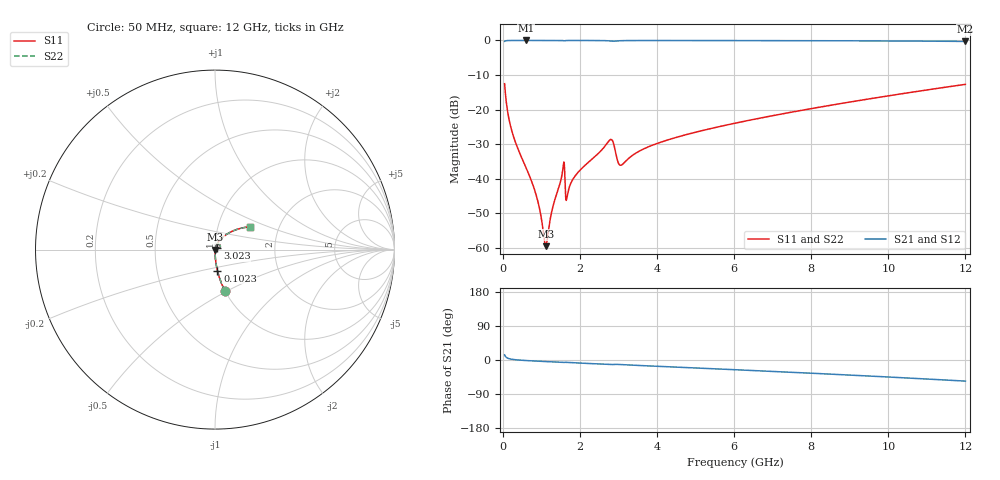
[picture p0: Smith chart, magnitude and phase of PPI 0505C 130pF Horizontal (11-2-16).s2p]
# MHz S MA R 50
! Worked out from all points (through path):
!   1601 points, 50 MHz to 12 GHz, reference 50 ohm
!   highest |S21| = -0.01 dB at 602.7 MHz (marker M1); lowest = -0.3 dB at 12 GHz (marker M2)
!   group delay of S21, straight-line fit = 13 ps
!   lowest |S11| = -59.5 dB at 1.118 GHz (marker M3), VSWR 1.00, Z = 50.1 - j0.00725 ohm
!   |S11| at or under -10 dB: start of sweep to end of sweep
!   |S22| runs from -59.5 to -12.5 dB; largest |S21 - S12| = 0
!   S11 on the Smith chart (normalised r, x): 50 MHz: 1.00, -0.49; 102.3 MHz: 1.00, -0.24; 3.023 GHz: 1.03, +0.02; 12 GHz: 1.42, +0.38
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50  0.237 -76.4  0.9712 13.5  0.9712 13.5  0.237 -76.4
102.2812  0.1177 -83.4  0.9927 6.4  0.9927 6.4  0.1177 -83.4
169.5  0.07032 -86.2  0.997 3.4  0.997 3.4  0.07032 -86.2
266.5938  0.04329 -87.8  0.9985 1.5  0.9985 1.5  0.04329 -87.8
602.6875  0.0146 -88.3  0.9991 -1.4  0.9991 -1.4  0.0146 -88.3
886.5  0.005378 -82.8  0.999 -3.0  0.999 -3.0  0.005378 -82.8
1073.219  0.001405 -46.1  0.9989 -3.9  0.9989 -3.9  0.001405 -46.1
1118.031  0.001065 -3.9  0.9989 -4.1  0.9989 -4.1  0.001065 -3.9
1162.844  0.001434 36.2  0.9988 -4.4  0.9988 -4.4  0.001434 36.2
1297.281  0.003858 67.1  0.9987 -5.0  0.9987 -5.0  0.003858 67.1
1543.75  0.0119 68.3  0.9967 -6.4  0.9967 -6.4  0.0119 68.3
1685.656  0.006134 63.1  0.9977 -6.6  0.9977 -6.6  0.006134 63.1
1820.094  0.009834 73.8  0.9983 -7.3  0.9983 -7.3  0.009834 73.8
2044.156  0.01404 75.1  0.9982 -8.4  0.9982 -8.4  0.01404 75.1
2791.031  0.03686 48.4  0.9812 -12.1  0.9812 -12.1  0.03686 48.4
2865.719  0.0337 28.5  0.9739 -11.8  0.9739 -11.8  0.0337 28.5
3022.562  0.01612 35.0  0.9887 -11.8  0.9887 -11.8  0.01612 35.0
4038.312  0.03296 69.1  0.9968 -16.7  0.9968 -16.7  0.03296 69.1
6025  0.06369 62.1  0.995 -25.6  0.995 -25.6  0.06369 62.1
8019.156  0.1039 53.4  0.9911 -34.9  0.9911 -34.9  0.1039 53.4
10013.31  0.1587 43.8  0.9831 -44.9  0.9831 -44.9  0.1587 43.8
12000  0.232 33.2  0.9676 -55.7  0.9676 -55.7  0.232 33.2
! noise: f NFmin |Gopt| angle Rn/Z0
50  0.0003874  0.8639  0.3351  0.0006107
1372  0.004214  0.6892  5.053  0.002632
2701  0.01534  0.8196  9.932  0.01769
4031  0.01001  0.6322  14.62  0.005035
5360  0.01162  0.5926  19.19  0.005094
6682  0.01365  0.5766  23.63  0.005624
8012  0.0158  0.5692  27.98  0.006267
9341  0.01805  0.5674  32.18  0.006996
1.067e+04  0.02044  0.5702  36.24  0.007828
1.2e+04  0.02301  0.5769  40.17  0.00879
